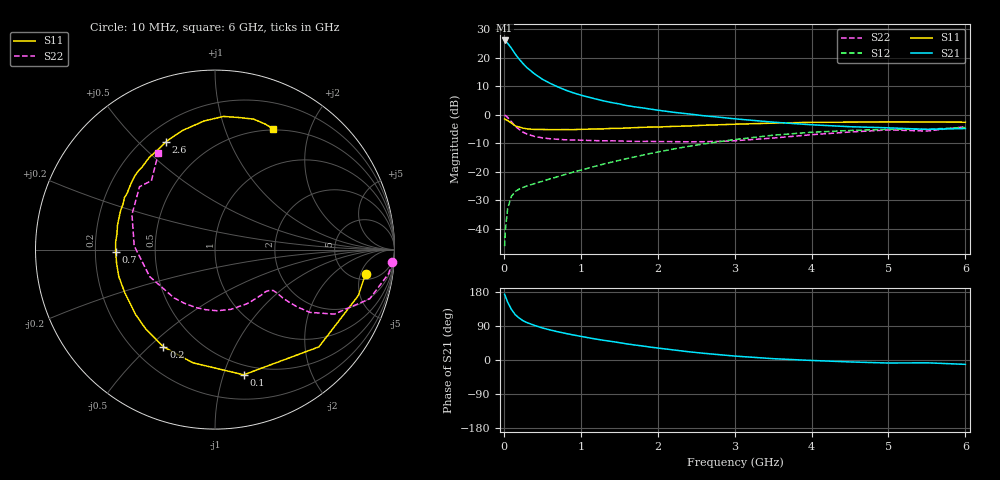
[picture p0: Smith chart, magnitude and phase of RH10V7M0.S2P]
! SIEMENS Small Signal Semiconductors
! BFR106
! Si NPN RF Bipolar Junction Transistor in SOT23
! VCE = 10 V  IC = 7 mA
! Common Emitter S-Parameters:  August  1996
# GHz  S  MA  R  50
!  f  S11  S21  S12  S22
! GHz  MAG  ANG  MAG  ANG  MAG  ANG  MAG  ANG
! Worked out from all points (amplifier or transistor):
!   36 points, 10 MHz to 6 GHz, reference 50 ohm
!   highest |S21| = 26.1 dB at 10 MHz (marker M1)
!   |S21| within 3 dB of that: start of sweep to 105.2 MHz
!   unconditionally stable (mu >= 1): 569.1 MHz to 1.889 GHz; 5.178 GHz to end of sweep
!   at 250 MHz: K = 0.59, MSG = 21.7 dB, |S12| = -25.4 dB
!   at 1.4 GHz: K = 1.11, MAG = 8.4 dB, |S12| = -16.6 dB
!   at 6 GHz: K = 1.01, MAG = -0.9 dB, |S12| = -4.4 dB
!   S11 on the Smith chart (normalised r, x): 10 MHz: 6.32, -6.13; 100 MHz: 0.41, -1.17; 200 MHz: 0.32, -0.55; 700 MHz: 0.29, -0.01; 2.6 GHz: 0.28, +0.61; 6 GHz: 0.49, +1.48
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0.01  0.8501 -9.1  20.27 173.4  0.005 88.3  0.9903 -3.9
0.02  0.8384 -17.8  19.89 168.4  0.0096 82.4  0.9773 -7.8
0.05  0.793 -43.1  18.08 152.3  0.0232 68.4  0.9049 -17.6
0.1  0.7157 -77.1  14.71 133.1  0.0377 55.5  0.7557 -28.4
0.15  0.6426 -101.0  11.62 119.2  0.0457 47.5  0.6335 -33.5
0.2  0.6132 -118.0  9.537 110.7  0.0501 45.0  0.557 -34.9
0.25  0.5871 -131.0  7.943 103.6  0.0538 43.3  0.4986 -35.4
0.3  0.5714 -140.6  6.773 98.8  0.0568 44.1  0.4635 -35.5
0.4  0.5569 -154.6  5.243 91.2  0.0627 46.2  0.4201 -35.0
0.5  0.5567 -164.3  4.243 84.7  0.0687 49.0  0.3965 -35.1
0.6  0.5536 -172.1  3.596 79.4  0.0757 51.6  0.3831 -36.3
0.7  0.5538 -178.9  3.117 74.6  0.0827 54.4  0.3742 -37.9
0.9  0.5532 170.8  2.45 66.2  0.0995 58.6  0.3637 -41.5
1.1  0.5634 161.6  2.054 58.7  0.117 61.5  0.3578 -47.2
1.3  0.5714 153.7  1.761 51.9  0.1383 63.1  0.3525 -53.0
1.6  0.5902 143.7  1.461 42.5  0.1719 64.0  0.3473 -63.4
2.2  0.6307 125.6  1.117 26.7  0.2522 60.8  0.3407 -88.2
2.6  0.6605 114.4  0.969 17.7  0.3102 56.0  0.3401 -108.3
3.5  0.7187 95.0  0.748 3.5  0.4417 41.2  0.3936 -157.5
4.5  0.7479 79.7  0.622 -5.1  0.5345 22.1  0.5022 157.1
5.5  0.7532 68.0  0.559 -7.4  0.5625 9.2  0.5224 132.7
6  0.7466 64.2  0.578 -11.5  0.6026 1.1  0.6214 120.5
